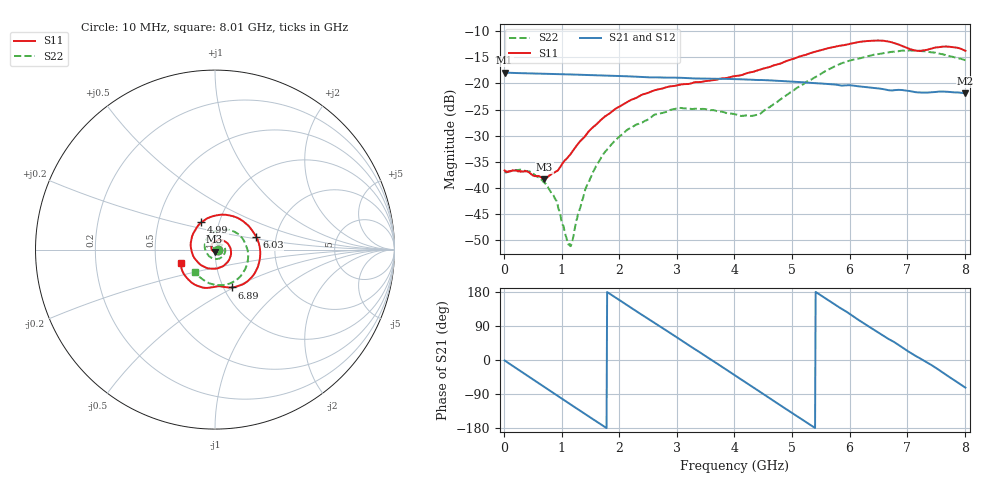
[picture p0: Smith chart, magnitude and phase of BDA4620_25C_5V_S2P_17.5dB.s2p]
!Agilent Technologies,E5071B,MY42404982,A.09.10
!Date: Wed May 06 09:01:59 2026
!Data & Calibration Information:
!Freq	S11:SOLT2(ON)	S21:SOLT2(ON)	S12:SOLT2(ON)	S22:SOLT2(ON)
# Hz S RI R 50
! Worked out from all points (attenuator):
!   801 points, 10 MHz to 8.01 GHz, reference 50 ohm
!   highest |S21| = -17.92 dB at 10 MHz (marker M1); lowest = -21.9 dB at 8.01 GHz (marker M2)
!   lowest |S11| = -38.3 dB at 700 MHz (marker M3), VSWR 1.02, Z = 49.7 - j1.18 ohm
!   |S11| at or under -10 dB: start of sweep to end of sweep
!   |S22| runs from -51.1 to -13.7 dB; largest |S21 - S12| = 0.00051
!   S11 on the Smith chart (normalised r, x): 10 MHz: 1.03, -0.00; 4.99 GHz: 0.82, +0.26; 6.03 GHz: 1.58, +0.23; 6.89 GHz: 1.09, -0.49; 8.01 GHz: 0.67, -0.11
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1e7  0.0147 -0.00101  0.127 -0.00268  0.1271 -0.00281  0.0141 -0.00051
4.2e8  0.00889 -0.0112  0.0914 -0.0854  0.0915 -0.0856  0.0134 -0.00524
7e8  -0.00272 -0.0119  0.0396 -0.1175  0.0396 -0.1177  0.00849 -0.00747
8.9e8  -0.0118 -0.00799  -0.00111 -0.1231  -0.00127 -0.1234  0.00342 -0.00707
1.14e9  -0.0198 0.00554  -0.0529 -0.11  -0.0531 -0.1101  -0.0024 -0.00164
1.19e9  -0.0205 0.00927  -0.0622 -0.1046  -0.0625 -0.1048  -0.00317 0.000109
1.35e9  -0.0202 0.0209  -0.0883 -0.0829  -0.0884 -0.0829  -0.00482 0.00549
1.58e9  -0.0113 0.0379  -0.1124 -0.0414  -0.1126 -0.0415  -0.00391 0.0149
1.87e9  0.0128 0.0521  -0.1171 0.0178  -0.1173 0.0179  0.00438 0.026
2.68e9  0.0879 0.000683  -0.00256 0.1142  -0.00238 0.1143  0.0472 0.019
3.41e9  0.0313 -0.0983  0.1055 0.0367  0.1057 0.0367  0.0443 -0.036
4.01e9  -0.0863 -0.0801  0.0834 -0.0716  0.0835 -0.0718  -0.014 -0.0489
4.42e9  -0.1342 0.00823  0.0159 -0.1067  0.0158 -0.1069  -0.0491 -0.0121
4.99e9  -0.0753 0.1521  -0.0783 -0.0688  -0.0784 -0.0689  -0.0344 0.0759
5.35e9  0.0334 0.1947  -0.1006 -0.00981  -0.1008 -0.00973  0.0245 0.1075
6.03e9  0.231 0.069  -0.0455 0.0843  -0.0456 0.0846  0.1574 0.056
6.36e9  0.2475 -0.066  0.00691 0.0909  0.00693 0.0909  0.1838 -0.017
6.68e9  0.1719 -0.1832  0.0492 0.0706  0.0493 0.0709  0.1733 -0.0963
6.89e9  0.0945 -0.2109  0.0706 0.0504  0.0708 0.0505  0.1465 -0.1439
7.19e9  0.0189 -0.2038  0.0813 0.00983  0.0817 0.0101  0.077 -0.191
7.57e9  -0.0862 -0.2059  0.0737 -0.0396  0.0739 -0.0396  -0.0223 -0.1905
8.01e9  -0.1912 -0.075  0.0236 -0.0768  0.0237 -0.077  -0.11 -0.125
